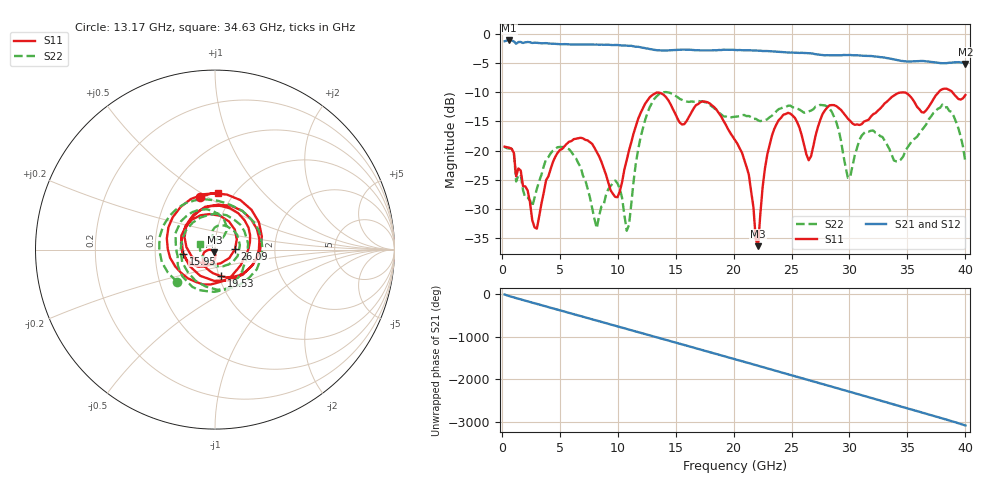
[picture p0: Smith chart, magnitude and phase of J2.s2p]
!Agilent Technologies,E8364B,MY43040528,A.07.50.67
!Agilent E8364B: A.07.50.67
!Date: Thursday, May 22, 2025 21:02:28
!Correction: S11(Full 2 Port(1,2))
!S21(Full 2 Port(1,2))
!S12(Full 2 Port(1,2))
!S22(Full 2 Port(1,2))
!S2P File: Measurements: S11, S21, S12, S22:
# Hz S  dB  R 50
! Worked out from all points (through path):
!   201 points, 250 MHz to 40 GHz, reference 50 ohm
!   highest |S21| = -1.12 dB at 647.5 MHz (marker M1); lowest = -5.1 dB at 40 GHz (marker M2)
!   group delay of S21, straight-line fit = 213 ps
!   lowest |S11| = -36.4 dB at 22.11 GHz (marker M3), VSWR 1.03, Z = 49.7 - j1.48 ohm
!   |S11| at or under -10 dB: start of sweep to 37.69 GHz; 38.88 GHz to end of sweep
!   |S22| runs from -33.7 to -10.0 dB; largest |S21 - S12| = 0.0064
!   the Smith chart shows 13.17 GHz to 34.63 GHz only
!   S11 on the Smith chart (normalised r, x): 13.17 GHz: 0.72, +0.47; 15.95 GHz: 0.70, -0.03; 19.53 GHz: 1.02, -0.31; 26.09 GHz: 1.25, +0.01; 34.63 GHz: 0.84, +0.59
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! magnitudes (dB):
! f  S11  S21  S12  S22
! 250 MHz  -19.3  -1.3  -1.3  -19.4
! 647.5 MHz  -19.5  -1.1  -1.1  -19.7
! 3.033 GHz  -33.4  -1.5  -1.5  -26.5
! 4.622 GHz  -21.0  -1.7  -1.7  -19.7
! 7.008 GHz  -17.9  -1.8  -1.8  -24.3
! 8.2 GHz  -20.2  -1.8  -1.8  -33.3
! 9.79 GHz  -27.9  -1.9  -1.9  -25.1
! 10.78 GHz  -21.6  -2.0  -2.0  -33.7
! 13.17 GHz  -10.3  -2.7  -2.7  -11.1
! 13.57 GHz  -10.1  -2.8  -2.8  -10.3
! 15.95 GHz  -14.9  -2.7  -2.7  -11.6
! 19.53 GHz  -16.3  -2.8  -2.7  -14.3
! 20.12 GHz  -18.2  -2.8  -2.8  -14.2
! 22.11 GHz  -36.4  -2.9  -2.9  -14.8
! 23.5 GHz  -16.3  -3.0  -3.0  -13.7
! 26.09 GHz  -19.1  -3.3  -3.3  -13.5
! 26.88 GHz  -19.2  -3.4  -3.4  -12.9
! 29.86 GHz  -14.5  -3.6  -3.6  -24.7
! 33.44 GHz  -11.2  -4.2  -4.3  -19.7
! 34.63 GHz  -10.0  -4.7  -4.7  -21.0
! 38.01 GHz  -9.5  -5.0  -5.0  -12.1
! 40 GHz  -10.5  -5.1  -5.1  -22.0
